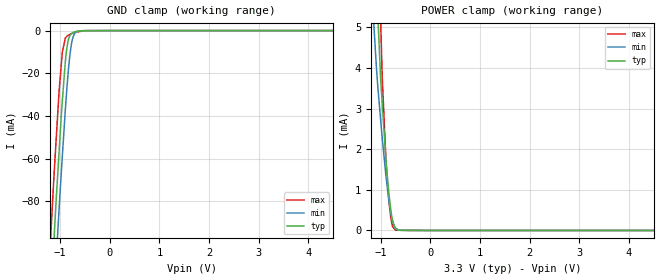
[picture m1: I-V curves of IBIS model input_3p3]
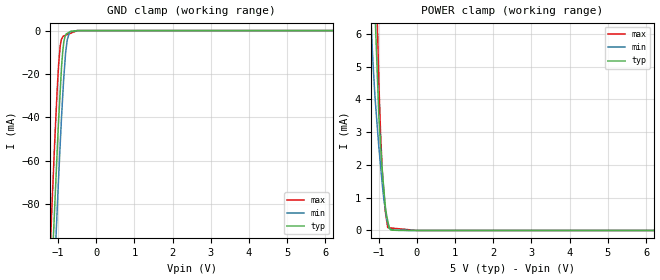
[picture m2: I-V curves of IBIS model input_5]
|Texas Instruments Incorporated
| 16-Bit, Ultra-Low Power, Voltage Output Digital to Analog Converter
| Marketing part#   Digital Voltage Range   Package-type   #pins
| DAC8831IBD   2.7V - 5.5V   SOIC   14
| DAC8831IBDG4   2.7V - 5.5V   SOIC   14
| DAC8831IBDR   2.7V - 5.5V   SOIC   14
| DAC8831IBDRG4   2.7V - 5.5V   SOIC   14
| DAC8831IBRGYR   2.7V - 5.5V   VQFN   14
| DAC8831IBRGYRG4   2.7V - 5.5V   VQFN   14
| DAC8831IBRGYT   2.7V - 5.5V   VQFN   14
| DAC8831IBRGYTG4   2.7V - 5.5V   VQFN   14
| DAC8831ICD   2.7V - 5.5V   SOIC   14
| DAC8831ICDG4   2.7V - 5.5V   SOIC   14
| DAC8831ICDR   2.7V - 5.5V   SOIC   14
| DAC8831ICDRG4   2.7V - 5.5V   SOIC   14
| DAC8831ICRGYR   2.7V - 5.5V   VQFN   14
| DAC8831ICRGYRG4   2.7V - 5.5V   VQFN   14
| DAC8831ICRGYT   2.7V - 5.5V   VQFN   14
| DAC8831ICRGYTG4   2.7V - 5.5V   VQFN   14
| DAC8831ID   2.7V - 5.5V   SOIC   14
| DAC8831IDG4   2.7V - 5.5V   SOIC   14
| DAC8831IDR   2.7V - 5.5V   SOIC   14
| DAC8831IDRG4   2.7V - 5.5V   SOIC   14
| DAC8831IRGYR   2.7V - 5.5V   VQFN   14
| DAC8831IRGYRG4   2.7V - 5.5V   VQFN   14
| DAC8831IRGYT   2.7V - 5.5V   VQFN   14
| DAC8831IRGYTG4   2.7V - 5.5V   VQFN   14
[IBIS Ver]   3.2
[File name]   dac8831.ibs
|SIMDE Ver   V3.0 - 201101 - RHL4 - Build 453
[File Rev]   1.0
[Date]   4/13/2011
[Source]
| Texas Instruments Incorporated.
| Analog-eLab Design Center, HPA
| 12500 TI Blvd
| Dallas, TX -75243
| e-mail: elab_ibis@list.ti.com
| -Model generated from simulations in TISPICE
[Notes]   Revision History:
| Rev 1.0: 4/13/2011
| - Initial version of the model
| - Model generated from simulations in TISPICE
| - Model matched to SPICE simulation
| - C_comp although listed in numerical order of value are
|   obtained from varying PVT conditions. For PVT conditions for
|   each specific value refer the buffer description under
|   respective [Model]. IBIS model user is responsible for using
|   appropriate C_comp to simulate for Signal Integrity.
| - Model names with a trailing _3p3 contains
|   the model for 3.3V [3.0V and 3.6V]. Model names with trailing _5
|   contains the model for 5.0V [4.5V and 5.5V] operation.
| - Relative of DAC8830.
[Disclaimer]
| This model is designed as an aid for customers of Texas Instruments.
| TI and its licensors and suppliers make no warranties, either expressed
| or implied, with respect to this  model, including the warranties of
| merchantability or fitness for a particular purpose. The model is
| provided solely on an "as is" basis. The entire risk as to its quality
| and performance is with the customer.
[Copyright]
 (C) Copyright 2011 Texas Instruments Incorporated.All rights reserved.
|   DAC8831D
[Component]   DAC8831D
[Manufacturer]   TI
[Package]   |14 SOIC   -  D package
|   typ   min   max
R_pkg   0.06973   0.04403   0.08357
L_pkg   2.62449nH   1.54367nH   3.39477nH
C_pkg   0.56417pF   0.37484pF   0.72997pF
[Pin]  signal_name   model_name   R_pin   L_pin   C_pin
1   RFB   TERM   0.08357   3.39477nH  0.72997pF
2   VOUT   TERM   0.07468   2.66777nH  0.56865pF
3   AGNDF   GND   0.03211   1.50207nH  0.41257pF
4   AGNDS   GND   0.04993   1.54725nH  0.37620pF
5   VREF-S   TERM   0.07562   2.15675nH  0.40446pF
6   VREF-F   TERM   0.04403   2.61165nH  0.60739pF
7   _CS   INPUT   0.07998   3.33489nH  0.71874pF
8   SCLK   INPUT   0.08026   3.34149nH  0.71730pF
9   NC   NC   0.00628   1.31996nH  0.47907pF
10   SDI   INPUT   0.06356   1.86895nH  0.38324pF
11   _LDAC   INPUT   0.04980   1.54367nH  0.37484pF
12   DGND   GND   0.07435   2.11708nH  0.40001pF
13   INV   TERM   0.07607   2.70047nH  0.57296pF
14   VDD   POWER   0.08034   3.31707nH  0.72723pF
|   DAC8831RGY
[Component]   DAC8831RGY
[Manufacturer]   TI
[Package]   |14 VQFN   -  RGY package
|   typ   min   max
R_pkg   0.03536   0.02104   0.04989
L_pkg   0.91851nH   0.72839nH   1.19016nH
C_pkg   0.12935pF   0.10533pF   0.15243pF
[Pin]  signal_name   model_name   R_pin   L_pin   C_pin
1   RFB   TERM   0.02532   0.94342nH  0.14951pF
2   VOUT   TERM   0.04989   1.19016nH  0.13397pF
3   AGNDF   GND   0.01883   0.61717nH  0.14816pF
4   AGNDS   GND   0.03684   0.84332nH  0.12234pF
5   VREF-S   TERM   0.04044   0.93565nH  0.13078pF
6   VREF-F   TERM   0.02254   0.80896nH  0.15243pF
7   _CS   INPUT   0.04370   1.02632nH  0.10927pF
8   SCLK   INPUT   0.04145   0.96430nH  0.10533pF
9   NC   NC   0.00040   0.06465nH  0.04885pF
10   SDI   INPUT   0.03694   0.83513nH  0.11768pF
11   _LDAC   INPUT   0.03692   0.83424nH  0.12018pF
12   DGND   GND   0.03985   0.91081nH  0.12690pF
13   INV   TERM   0.02104   0.72839nH  0.14503pF
14   VDD   POWER   0.04276   0.99343nH  0.09808pF
|   Model Selectors
[Model Selector] INPUT
input_3p3  3.3V digital input
input_5   5.0V digital input
[Model Selector] TERM
term_3-3V  3.3V nominal termination
term_5-0V  5.0V nominal termination
[Model]  term_3-3V
Model_type Terminator
C_comp   1.0e-20F  1.0e-20F  1.0e-20F
|   typ   min   max
[Voltage Range]   3.3V   3.0V   3.6V
[POWER Clamp Reference]   3.3V   3.0V   3.6V
[GND Clamp Reference]   0V   0V   0V
|Ambient Temperature   25   85   -40
|Junction Temperature
[Temperature Range]   28   88   -40
[Model]  term_5-0V
Model_type Terminator
C_comp   1.0e-20F  1.0e-20F  1.0e-20F
|   typ   min   max
[Voltage Range]   5.0V   4.5V   5.5V
[POWER Clamp Reference]   5.0V   4.5V   5.5V
[GND Clamp Reference]   0V   0V   0V
|Ambient Temperature   25   85   -40
|Junction Temperature
[Temperature Range]   28   88   -40
| Models and submodels in the file (4): input_3p3 (Input), input_5 (Input), term_3-3V (Terminator), term_5-0V (Terminator)
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|   input_3p3 Model
[Model]   input_3p3
Model_type   Input
Vinl = 0.6
Vinh = 2.1
|   typ   min   max
|   (nom PVT)   (Fast PVT)   (slow PVT)
|C_comp from frequency method(F=50MHz)
|Average
|C_comp   1.138e-12   1.128e-12   1.164e-12
|C_comp from L-C Tank method(L=1nH)
|Resonant Frequency(Hz)   5.500e9   5.670e9   5.310e9
C_comp   8.382e-13   7.887e-13   8.993e-13
| Where nom  PVT is Nominal Process,  3.3V,  28C
|   Fast PVT is Strong Process,   3.6V,  -40C
|   Slow PVT is Weak Process,   3V,  88C
[Voltage Range]   3.3   3   3.6
|Ambient Temperature   25   85   -40
|Junction Temperature
[Temperature Range]   28   88   -40
[Power Clamp Reference]   3.3   3   3.6
[GND Clamp Reference]   0   0   0
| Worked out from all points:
|   GND clamp passes 1 mA (typ) near -0.75 V on its own axis
|   POWER clamp passes 1 mA (typ) near -0.84 V on its own axis
[GND Clamp]
|   Voltage   I(typ)   I(min)   I(max)
-3.3V     -1.089A    -1.108A    -1.071A
-1.247V   -149.3mA   -177.7mA   -120.6mA
-1.138V   -103mA     -130.8mA   -73.2mA
-1.116V   -93.89mA   -121.6mA   -64.29mA
-1.082V   -79.77mA   -107.9mA   -51.4mA
-1.026V   -58.15mA   -84.95mA   -29.74mA
-957.6mV  -33.16mA   -59.12mA   -10.16mA
-881.1mV  -11.05mA   -32.01mA   -3.099mA
-807mV    -2.494mA   -11.97mA   -1.828mA
-726mV    -734.6uA   -2.062mA   -1.006mA
-441mV    -112.5uA   -2.337uA   -2.215uA
6.6V      0A         0A         0A
[POWER Clamp]
|   Voltage   I(typ)   I(min)   I(max)
-3.3V     114.7mA    94.01mA    143.3mA
-1.161V   9.141mA    5.478mA    13.29mA
-1.092V   6.393mA    4.078mA    9.463mA
-1.051V   5.046mA    3.4mA      7.199mA
-1.003V   3.718mA    2.717mA    5.129mA
-972mV    3.133mA    2.273mA    3.784mA
-896.4mV  1.722mA    1.341mA    1.708mA
-874.8mV  1.419mA    1.113mA    1.312mA
-828mV    819.7uA    645.8uA    629.4uA
-792mV    444.8uA    376.3uA    264.9uA
-702mV    41uA       57.9uA     7.242uA
6.6V      0A         0A         0A
|   input_5 Model
[Model]   input_5
Model_type   Input
Vinl = 0.8
Vinh = 2.4
|   typ   min   max
|   (nom PVT)   (Fast PVT)   (slow PVT)
|C_comp from frequency method(F=50MHz)
|Average
|C_comp   1.055e-12   1.045e-12   1.082e-12
|C_comp from L-C Tank method(L=1nH)
|Resonant Frequency(Hz)   5.630e9   5.750e9   5.460e9
C_comp   7.999e-13   7.669e-13   8.505e-13
| Where nom  PVT is Nominal Process,  5V,  28C
|   Fast PVT is Strong Process,   5.5V,  -40C
|   Slow PVT is Weak Process,   4.5V,  88C
[Voltage Range]   5   4.5   5.5
|Ambient Temperature   25   85   -40
|Junction Temperature
[Temperature Range]   28   88   -40
[Power Clamp Reference]   5   4.5   5.5
[GND Clamp Reference]   0   0   0
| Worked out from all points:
|   GND clamp passes 1 mA (typ) near -0.73 V on its own axis
|   POWER clamp passes 1 mA (typ) near -0.84 V on its own axis
[GND Clamp]
|   Voltage   I(typ)   I(min)   I(max)
-5V       -1.88A     -1.895A    -1.869A
-1.215V   -135.4mA   -163.4mA   -106.7mA
-1.14V    -103.5mA   -131.9mA   -74.27mA
-1.078V   -78.9mA    -106mA     -49.08mA
-1.023V   -57.05mA   -84.03mA   -28.71mA
-979mV    -40.41mA   -66.71mA   -15.14mA
-940.5mV  -28.05mA   -52.25mA   -7.211mA
-875mV    -9.833mA   -30.28mA   -2.936mA
-796.5mV  -2.074mA   -9.922mA   -2.147mA
-756mV    -1.287mA   -4.245mA   -1.86mA
-670mV    -370.3uA   -532.4uA   -1.251mA
10V       0A         0A         0A
[POWER Clamp]
|   Voltage   I(typ)   I(min)   I(max)
-5V       201mA      168.6mA    248.1mA
-1.215V   11.3mA     6.9mA      15.99mA
-1.161V   9.059mA    5.478mA    12.98mA
-1.089V   6.563mA    4.011mA    9.096mA
-1.056V   5.513mA    3.512mA    7.433mA
-990mV    3.412mA    2.514mA    4.467mA
-946mV    2.604mA    1.96mA     2.925mA
-907.5mV  1.898mA    1.476mA    1.939mA
-825mV    774.8uA    662.3uA    593.1uA
-759mV    295.2uA    233.4uA    84.34uA
-670mV    11.75uA    25.5uA     74.45uA
10V       0A         0A         0A
